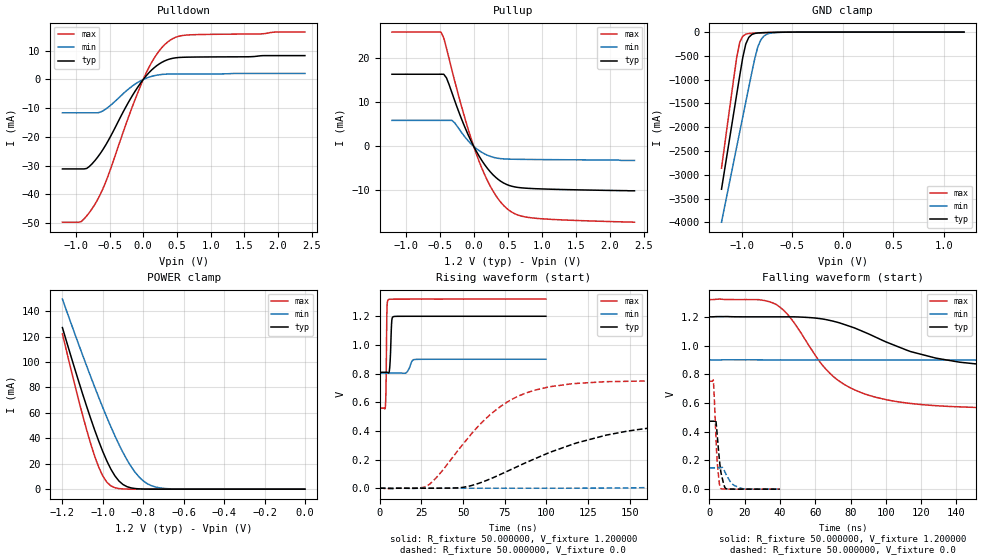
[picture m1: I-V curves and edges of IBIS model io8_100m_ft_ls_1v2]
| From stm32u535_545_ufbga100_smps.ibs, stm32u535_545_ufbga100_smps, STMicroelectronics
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|   Model io8_100m_ft_ls_1v2
[Model]  io8_100m_ft_ls_1v2
Model_type I/O
Polarity   Non-Inverting
Enable   Active-Low
Vinl =   0.360000V
Vinh =   0.840000V
Vmeas =  0.600000V
Cref =   50.000000pF
Rref =   100.000000M
Vref =   0.0V
C_comp   2.947800pF   2.877700pF   2.996100pF
[Temperature Range]   25.000000   0.140000k   -40.000000
[Pullup Reference]   1.200000V   0.900000V   1.320000V
[Pulldown Reference]   0.0V   0.0V   0.0V
[POWER Clamp Reference]   1.200000V   0.900000V   1.320000V
[GND Clamp Reference]   0.0V   0.0V   0.0V
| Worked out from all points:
|   slope of the pulldown table from 0 to 0.18 V, typ, clamps not added: 40.7 ohm
|   slope of the pullup table from 0 to 0.18 V, typ, clamps not added: 39.5 ohm
|   GND clamp passes 1 mA (typ) near -0.51 V on its own axis
|   POWER clamp passes 1 mA (typ) near -0.86 V on its own axis
|   rising waveform, R_fixture 50.000000, V_fixture 1.200000: 20-80 % time 754ps typ, 2.06ns min, 442ps max; typ from 0.809 V to 1.2 V
|   rising waveform, R_fixture 50.000000, V_fixture 0.0: 20-80 % time 67.4ns typ, 166ns min, 37.1ns max; typ from 0 V to 0.473 V
|   falling waveform, R_fixture 50.000000, V_fixture 1.200000: 20-80 % time 57.9ns typ, 150ns min, 31.6ns max; typ from 1.2 V to 0.809 V
|   falling waveform, R_fixture 50.000000, V_fixture 0.0: 20-80 % time 2.49ns typ, 4.76ns min, 1.84ns max; typ from 0.473 V to 0 V
[Pulldown]
|Voltage   I(typ)   I(min)   I(max)
-1.2V     -31.16mA   -11.61mA   -49.71mA
-920mV    -31.16mA   -11.61mA   -49.48mA
-840mV    -31mA      -11.61mA   -47.54mA
-720mV    -28.32mA   -11.61mA   -43.58mA
-560mV    -22.95mA   -10.37mA   -35.89mA
-200mV    -7.146mA   -2.964mA   -11.89mA
0V        0A         0A         0A
160mV     4.047mA    1.298mA    7.361mA
360mV     6.87mA     1.87mA     13mA
480mV     7.543mA    1.91mA     14.69mA
640mV     7.764mA    1.923mA    15.46mA
2.4V      8.308mA    2.101mA    16.5mA
[Pullup]
|Voltage   I(typ)   I(min)   I(max)
-1.2V     16.39mA    5.9mA      25.96mA
-480mV    16.39mA    5.9mA      25.96mA
-440mV    16.39mA    5.9mA      24.63mA
-400mV    15.57mA    5.9mA      22.35mA
-320mV    12.21mA    5.9mA      17.37mA
-120mV    3.997mA    1.962mA    5.905mA
80mV      -2.237mA   -962.6uA   -3.434mA
280mV     -6.404mA   -2.453mA   -10.06mA
520mV     -8.88mA    -2.901mA   -14.54mA
680mV     -9.389mA   -2.951mA   -15.76mA
920mV     -9.627mA   -2.991mA   -16.35mA
2.36V     -10.1mA    -3.2mA     -17.23mA
[GND_clamp]
|Voltage   I(typ)   I(min)   I(max)
-1.2V     -3.305A    -3.998A    -2.862A
-1.05V    -1.316A    -2.418A    -539.3mA
-1.02V    -921mA     -2.103A    -218.8mA
-990mV    -539.5mA   -1.788A    -87.43mA
-960mV    -252.1mA   -1.474A    -44.36mA
-930mV    -110.5mA   -1.16A     -30.32mA
-870mV    -28.03mA   -549.1mA   -21.09mA
-840mV    -18.43mA   -305.6mA   -18.27mA
-810mV    -13.9mA    -159.7mA   -15.73mA
-780mV    -11.23mA   -82.35mA   -13.37mA
-600mV    -2.976mA   -4.272mA   -3.058mA
1.2V      0A         14.74nA    0A
[POWER_clamp]
|Voltage   I(typ)   I(min)   I(max)
-1.2V     127mA      149.4mA    122.2mA
-1.12V    84.97mA    114mA      70.27mA
-1.06V    55.51mA    88.42mA    35.67mA
-1.02V    37.63mA    72.04mA    17.17mA
-1V       29.51mA    64.13mA    10.3mA
-960mV    15.69mA    48.99mA    2.571mA
-900mV    3.624mA    28.77mA    182.8uA
-840mV    490.7uA    13.24mA    11.35uA
-800mV    116.8uA    6.532mA    1.77uA
-740mV    13.2uA     1.723mA    109.1nA
-620mV    167.3nA    79.35uA    0A
0V        0A         17.84nA    0A
[Ramp]
| variable   typ   min   max
dV/dt_r  0.28373/67.34885n   88.87787m/0.16576u  0.45090/37.03275n
dV/dt_f  0.23462/57.84131n   57.86400m/0.14950u  0.45665/31.51629n
R_load = 50.000000
[Rising Waveform]
R_fixture= 50.000000
V_fixture= 1.200000
V_fixture_min= 0.900000
V_fixture_max= 1.320000
|time   V(typ)   V(min)   V(max)
0s        809mV      803.5mV    558.9mV
3.403ns   809mV      803.5mV    575.3mV
3.804ns   809.1mV    803.5mV    765.4mV
4.204ns   809mV      803.5mV    1.213V
5.205ns   804.5mV    803.5mV    1.317V
6.006ns   852.7mV    803.5mV    1.319V
7.207ns   1.173V     803.5mV    1.319V
8.208ns   1.197V     803.5mV    1.319V
21.02ns   1.2V       898.3mV    1.32V
99.7ns    1.2V       900mV      1.32V
[Rising Waveform]
R_fixture= 50.000000
V_fixture= 0.0
V_fixture_min= 0.0
V_fixture_max= 0.0
|time   V(typ)   V(min)   V(max)
0s        2.277nV    212.1nV    1.455nV
28.03ns   -93.62uV   -27.51uV   14.01mV
50.05ns   6.457mV    -22uV      309.3mV
72.07ns   94.67mV    16.68uV    567.2mV
92.09ns   200.6mV    68.91uV    681mV
116.1ns   308.3mV    372.9uV    729.9mV
166.2ns   425.1mV    5.867mV    749.6mV
246.2ns   467.4mV    49.17mV    751.6mV
462.5ns   472.9mV    136.2mV    751.5mV
997ns     472.9mV    148.2mV    751.6mV
[Falling Waveform]
R_fixture= 50.000000
V_fixture= 1.200000
V_fixture_min= 0.900000
V_fixture_max= 1.320000
|time   V(typ)   V(min)   V(max)
0s        1.2V       900mV      1.32V
36.04ns   1.2V       900.1mV    1.296V
46.05ns   1.2V       900mV      1.191V
64.06ns   1.185V     900mV      863.4mV
76.08ns   1.148V     900mV      732mV
98.1ns    1.036V     900mV      628.9mV
128.1ns   913.1mV    899.6mV    581.4mV
246.2ns   816.3mV    866.8mV    559.1mV
444.4ns   809.1mV    812.9mV    558.9mV
997ns     809mV      803.5mV    558.9mV
[Falling Waveform]
R_fixture= 50.000000
V_fixture= 0.0
V_fixture_min= 0.0
V_fixture_max= 0.0
|time   V(typ)   V(min)   V(max)
0s        472.9mV    148.2mV    751.6mV
2.242ns   472.9mV    148.2mV    756.4mV
3.604ns   480.1mV    148.2mV    396.4mV
4.324ns   393.9mV    148.2mV    212.3mV
5.606ns   215.4mV    148mV      44.36mV
6.166ns   151.1mV    148.4mV    8.929mV
8.008ns   40.03mV    140.5mV    1.16mV
9.369ns   3.165mV    106.1mV    423.4uV
17.22ns   38.23uV    8.44mV     -19.19uV
39.88ns   2.277nV    212.1nV    1.455nV
